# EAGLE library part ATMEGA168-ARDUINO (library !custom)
ATmega168/328 Arduino Pin Map. Dual In Line (DIL) 28 pin IC at standard 600mil spacing.
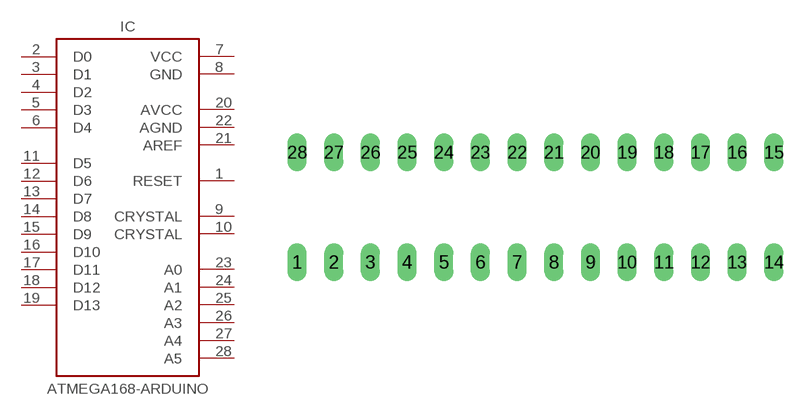
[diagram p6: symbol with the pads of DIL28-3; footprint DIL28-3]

Designator prefix IC

## ATMEGA168-ARDUINO  [DIL28-3]
1  RESET  pas
2  D0  pas
3  D1  pas
4  D2  pas
5  D3  pas
6  D4  pas
7  VCC  pas
8  GND  pas
9  CRYSTAL  pas
10  CRYSTAL  pas
11  D5  pas
12  D6  pas
13  D7  pas
14  D8  pas
15  D9  pas
16  D10  pas
17  D11  pas
18  D12  pas
19  D13  pas
20  AVCC  pas
21  AREF  pas
22  AGND  pas
23  A0  pas
24  A1  pas
25  A2  pas
26  A3  pas
27  A4  pas
28  A5  pas

## Footprint DIL28-3 (pad centres in mm)
Dual In Line 0.3 inch
drill 0.813 long: 1 -16.51,-3.81; 2 -13.97,-3.81; 3 -11.43,-3.81; 4 -8.89,-3.81; 5 -6.35,-3.81; 6 -3.81,-3.81; 7 -1.27,-3.81; 8 1.27,-3.81; 9 3.81,-3.81; 10 6.35,-3.81; 11 8.89,-3.81; 12 11.43,-3.81; 13 13.97,-3.81; 14 16.51,-3.81; 15 16.51,3.81; 16 13.97,3.81; 17 11.43,3.81; 18 8.89,3.81; 19 6.35,3.81; 20 3.81,3.81; 21 1.27,3.81; 22 -1.27,3.81; 23 -3.81,3.81; 24 -6.35,3.81; 25 -8.89,3.81; 26 -11.43,3.81; 27 -13.97,3.81; 28 -16.51,3.81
